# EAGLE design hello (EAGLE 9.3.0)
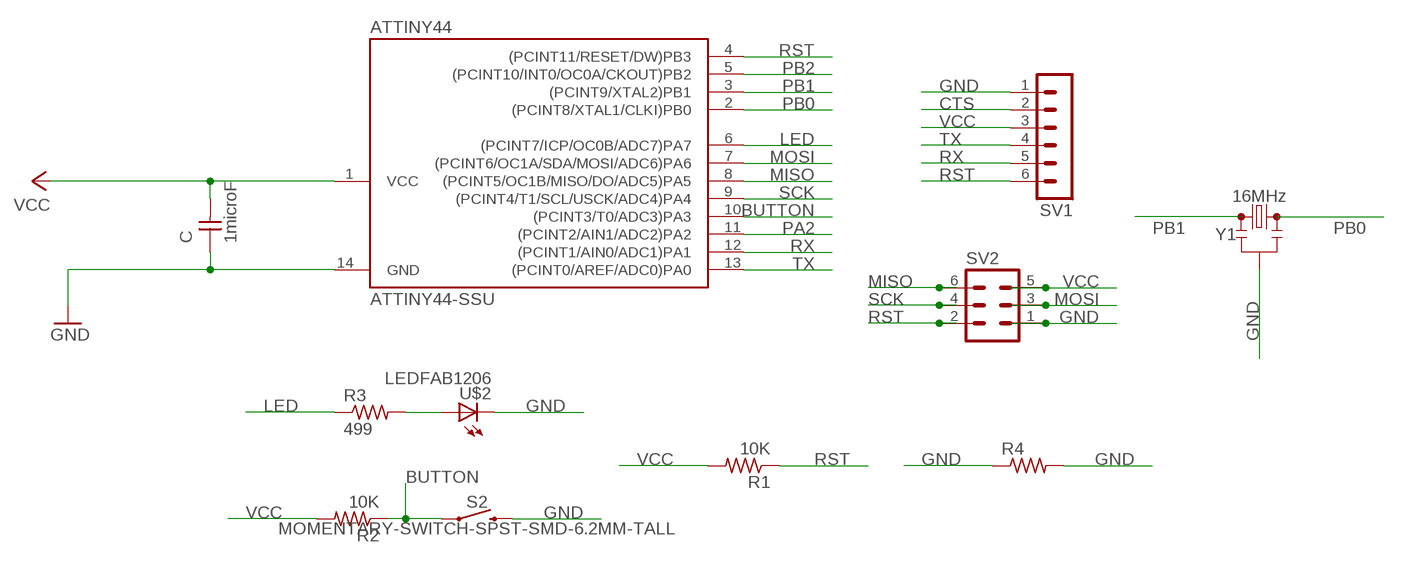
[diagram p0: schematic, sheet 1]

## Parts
ATTINY44  ATTINY44-SSU  [SOIC14]
C  1microF  CAP-UNPOLARIZED  [C1206]
R1  10K  RES-US1206FAB  [R1206FAB]
R2  10K  RES-US1206FAB  [R1206FAB]
R3  499  RES-US1206FAB  [R1206FAB]
R4  RES-US1206FAB  [R1206FAB]
S2  MOMENTARY-SWITCH-SPST-SMD-6.2MM-TALL  [TACTILE_SWITCH_SMD_6.2MM_TALL]
SV1  MA06-1  [MA06-1]
SV2  MA03-2  [MA03-2]
U$2  LEDFAB1206  [LED1206FAB]
Y1  16MHz  RESONATOR-16MHZSMD_3.2X1.3  [RESONATOR-SMD-3.2X1.3]

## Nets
BUTTON: ATTINY44.10((PCINT3/T0/ADC3)PA3) R2.1 S2.A2
CTS: SV1.2
GND: ATTINY44.14(GND) C.1 R4.1 R4.2 S2.B2 SV1.1 SV2.1 U$2.2(C) Y1.2
LED: ATTINY44.6((PCINT7/ICP/OC0B/ADC7)PA7) R3.1
MISO: ATTINY44.8((PCINT5/OC1B/MISO/DO/ADC5)PA5) SV2.6
MOSI: ATTINY44.7((PCINT6/OC1A/SDA/MOSI/ADC6)PA6) SV2.3
N$1: R3.2 U$2.1(A)
PA2: ATTINY44.11((PCINT2/AIN1/ADC2)PA2)
PB0: ATTINY44.2((PCINT8/XTAL1/CLKI)PB0) Y1.3
PB1: ATTINY44.3((PCINT9/XTAL2)PB1) Y1.1
PB2: ATTINY44.5((PCINT10/INT0/OC0A/CKOUT)PB2)
RST: ATTINY44.4((PCINT11/RESET/DW)PB3) R1.1 SV1.6 SV2.2
RX: ATTINY44.12((PCINT1/AIN0/ADC1)PA1) SV1.5
SCK: ATTINY44.9((PCINT4/T1/SCL/USCK/ADC4)PA4) SV2.4
TX: ATTINY44.13((PCINT0/AREF/ADC0)PA0) SV1.4
VCC: ATTINY44.1(VCC) C.2 R1.2 R2.2 SV1.3 SV2.5

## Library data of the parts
ATTINY44 = fab:ATTINY44
C = fab:CAP-UNPOLARIZED
R1-R4 = fab:RES-US: Resistor (US Symbol)
S2 = SparkFun-Switches:MOMENTARY-SWITCH-SPST: Momentary Switch (Pushbutton) - SPST; PROD_ID: SWCH-11966; SF_SKU: COM-12992
SV1 = con-lstb:MA06-1: PIN HEADER; OC_FARNELL: unknown; OC_NEWARK: unknown
SV2 = con-lstb:MA03-2: PIN HEADER; OC_FARNELL: unknown; OC_NEWARK: unknown
U$2 = fab:LED: LED
Y1 = SparkFun-Clocks:RESONATOR-16MHZ: 16MHz Resonator Digikey Example Frequency: 16MHz Frequency Stability: &plusmn;0.3% Frequency Tolerance: &plusmn;0.5% Capacitance: 15pF SparkFun Products SparkFun OpenLog SparkFun MicroView - OLED Arduino Module; PROD_ID: XTAL-08900

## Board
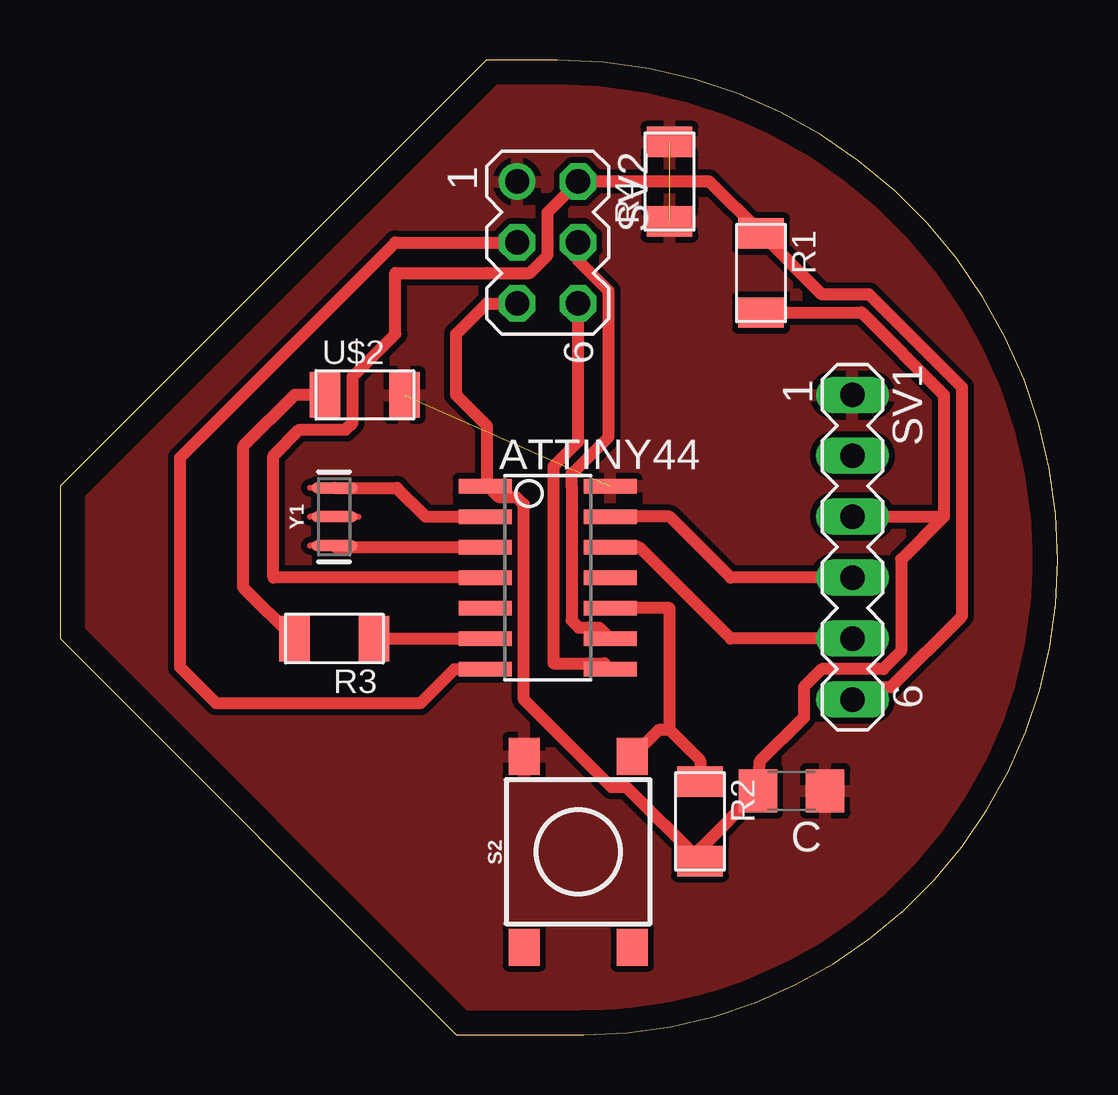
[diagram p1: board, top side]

Size 41.58 x 40.63 mm. Coordinates in mm from the lower left corner, seen from the top.
Outline: 0,22.86 0,16.51 16.51,0 21.81,0 arc90 41.58,19.77 arc90 20.72,40.63 17.77,40.63 0,22.86
Copper layers (1*16): Top 0.035mm / dielectric 1.5mm / Bottom 0.035mm
Design rules "default *": minimum track width 0.2mm, minimum drill 0.35mm, track to track 0.25mm, track to pad 0.25mm, pad to pad 0.25mm, via to via 0.25mm, smd to smd 0.25mm, copper to edge 40mil, drill to drill 6mil, minimum pad ring 10mil, minimum via ring 8mil, stop-mask expansion 4mil, vias tented up to drill 0mil, thermal gap 10mil

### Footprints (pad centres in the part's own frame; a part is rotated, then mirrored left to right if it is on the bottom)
SOIC14 = smd 0.61 x 2.21: 1 -3.81,-2.603; 2 -2.54,-2.603; 3 -1.27,-2.603; 4 0,-2.603; 5 1.27,-2.603; 6 2.54,-2.603; 7 3.81,-2.603; 8 3.81,2.603; 9 2.54,2.603; 10 1.27,2.603; 11 0,2.603; 12 -1.27,2.603; 13 -2.54,2.603; 14 -3.81,2.603
C1206 = smd 1.6 x 1.8: 1 -1.4,0; 2 1.4,0
R1206FAB = smd 1.27 x 1.905: 1 -1.651,0; 2 1.651,0
TACTILE_SWITCH_SMD_6.2MM_TALL = smd 1.55 x 1.3: A1 -3.975,-2.25; A2 3.975,-2.25; B1 -3.975,2.25; B2 3.975,2.25
MA06-1 = drill 1.016 long: 1 -6.35,0; 2 -3.81,0; 3 -1.27,0; 4 1.27,0; 5 3.81,0; 6 6.35,0
MA03-2 = drill 1.016: 1 -2.54,-1.27 | drill 1.016 octagon: 2 -2.54,1.27; 3 0,-1.27; 4 0,1.27; 5 2.54,-1.27; 6 2.54,1.27
LED1206FAB = smd 1.27 x 1.905: 1 -1.651,0; 2 1.651,0
RESONATOR-SMD-3.2X1.3 = smd 0.45 x 1.905: 1 -1.2,0; 2 0,0; 3 1.2,0

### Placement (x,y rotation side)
ATTINY44  20.32,19.05 270 top
C  30.48,10.16 180 top
R1  29.21,31.75 270 top
R2  26.67,8.89 270 top
R3  11.43,16.51 180 top
R4  25.4,35.56 90 top
S2  21.59,7.62 90 top
SV1  33.02,20.32 270 top
SV2  20.32,33.02 270 top
U$2  12.7,26.67 0 top
Y1  11.43,21.59 90 top

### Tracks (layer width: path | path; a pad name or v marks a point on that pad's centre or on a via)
BUTTON
  Top 0.508: ATTINY44.10 25.4,17.78 25.4,12.7 | 25.4,12.7 26.67,11.43 R2.1 | 25.4,12.7 24.95,12.7 S2.A2
GND  (2 unrouted)
  Top 0.508: 13.97,27.05 U$2.2
  pour Top: 17.78,46.99 arc90 -15.24,13.97 arc90 -1.27,0 29.21,0 arc90 46.99,17.78 arc90
LED
  Top 0.508: R3.1 ATTINY44.6
MISO
  Top 0.508: SV2.6 21.59,24.72 20.56,23.69 20.56,15.48 22.69,15.48 ATTINY44.8
MOSI
  Top 0.508: ATTINY44.7 16.45,15.24 15.02,13.82 6.5,13.82 4.99,15.33 4.99,24.04 13.97,33.02 SV2.3
N$1
  Top 0.508: 11.43,26.29 U$2.1 9.78,26.67 7.62,24.51 7.62,18.67 R3.2
PB0
  Top 0.508: Y1.3 14.04,22.79 15.24,21.59 ATTINY44.2
PB1
  Top 0.508: Y1.1 11.5,20.32 ATTINY44.3
RST
  Top 0.508: ATTINY44.4 8.89,19.05 8.89,24.13 9.97,25.21 11.89,25.21 12.19,25.51 12.19,27.43 13.97,29.21 13.97,31.75 17.78,31.75 19.57,31.75 20.32,32.5 20.32,34.29 SV2.2 27.05,35.56 R1.1 31.75,30.86 33.71,30.86 37.59,26.98 37.59,17.45 34.62,14.49 33.54,14.49 SV1.6
RX
  Top 0.508: ATTINY44.12 24.13,20.32 27.94,16.51 SV1.5
SCK
  Top 0.508: 22.21,16.51 ATTINY44.9 22.46,16.97 21.61,16.97 21.31,17.27 21.31,22.86 21.31,23.37 22.86,24.91 22.86,31 21.59,32.27 SV2.4
TX
  Top 0.508: SV1.4 27.94,19.05 25.4,21.59 ATTINY44.13
VCC
  Top 0.508: 17.78,22.92 17.78,25.4 16.51,26.67 16.51,29.21 17.78,30.48 SV2.5 | 17.78,22.92 ATTINY44.1 | 36.83,21.59 SV1.3 31.75,21.59 | R1.2 33.4,30.1 36.83,26.67 36.83,21.59 | 36.83,21.59 35.05,19.81 35.05,15.99 34.31,15.24 31.74,15.24 30.99,14.49 30.99,13.21 29.14,11.36 C.2 26.67,7.75 R2.2 23.59,10.32 22.98,10.32 19.33,13.97 19.33,22.1 19.03,22.4 18.3,22.4 17.78,22.92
